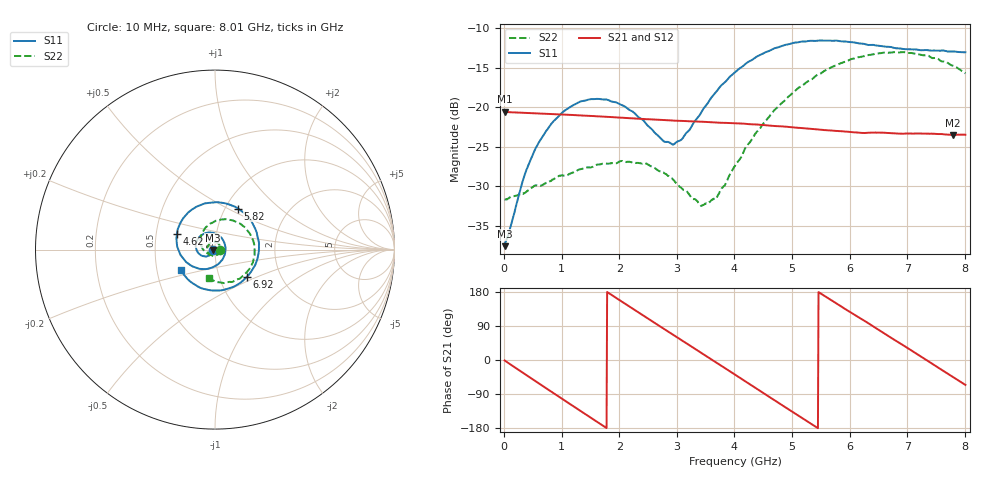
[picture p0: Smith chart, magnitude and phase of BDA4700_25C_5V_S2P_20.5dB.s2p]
!Agilent Technologies,E5071B,MY42404982,A.09.10
!Date: Mon Oct 20 13:36:39 2025
!Data & Calibration Information:
!Freq	S11:SOLT2(ON)	S21:SOLT2(ON)	S12:SOLT2(ON)	S22:SOLT2(ON)
# Hz S RI R 50
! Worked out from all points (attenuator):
!   801 points, 10 MHz to 8.01 GHz, reference 50 ohm
!   highest |S21| = -20.59 dB at 10 MHz (marker M1); lowest = -23.5 dB at 7.8 GHz (marker M2)
!   lowest |S11| = -37.6 dB at 10 MHz (marker M3), VSWR 1.03, Z = 48.7 - j0.149 ohm
!   |S11| at or under -10 dB: start of sweep to end of sweep
!   |S22| runs from -32.5 to -13.0 dB; largest |S21 - S12| = 0.00076
!   S11 on the Smith chart (normalised r, x): 10 MHz: 0.97, -0.00; 4.62 GHz: 0.64, +0.12; 5.82 GHz: 1.15, +0.56; 6.92 GHz: 1.36, -0.43; 8.01 GHz: 0.66, -0.16
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1e7  -0.0131 -0.00153  0.0935 -0.00199  0.0934 -0.00208  0.026 -0.000801
3.5e8  -0.0246 -0.0269  0.0745 -0.0541  0.0745 -0.0542  0.0222 -0.0178
5.7e8  -0.0427 -0.0376  0.0481 -0.0777  0.048 -0.0777  0.0143 -0.0286
8.8e8  -0.0763 -0.0328  0.000796 -0.0902  0.000764 -0.0904  -0.00699 -0.0347
1.35e9  -0.1077 0.0183  -0.0644 -0.0608  -0.0645 -0.0608  -0.0366 -0.0176
1.98e9  -0.052 0.0923  -0.0811 0.0287  -0.0811 0.0287  -0.0337 0.0294
2.46e9  0.0265 0.0746  -0.0331 0.0772  -0.0331 0.0772  -0.00135 0.0439
2.68e9  0.0511 0.0414  -0.00233 0.0832  -0.00236 0.0832  0.0141 0.0371
2.97e9  0.0567 -0.016  0.0369 0.0733  0.037 0.0732  0.0265 0.0206
3.44e9  -0.00467 -0.0948  0.0772 0.024  0.0773 0.024  0.0182 -0.0154
3.69e9  -0.064 -0.1081  0.0793 -0.01  0.0794 -0.0102  -0.000326 -0.0267
4.01e9  -0.1448 -0.0811  0.0618 -0.0494  0.0618 -0.0494  -0.0334 -0.0262
4.62e9  -0.2119 0.0852  -0.0117 -0.0755  -0.0117 -0.0755  -0.0797 0.0392
4.94e9  -0.1695 0.1844  -0.0483 -0.0573  -0.0483 -0.0575  -0.0712 0.0926
5.35e9  -0.0442 0.2591  -0.0718 -0.0124  -0.0718 -0.0126  -0.015 0.1498
5.82e9  0.1281 0.2285  -0.0575 0.0409  -0.0574 0.041  0.0908 0.1643
6.24e9  0.2301 0.1025  -0.0177 0.0664  -0.0171 0.0666  0.1802 0.1073
6.68e9  0.2305 -0.0698  0.0317 0.0609  0.0318 0.0609  0.2214 -0.00295
6.92e9  0.1792 -0.1499  0.0523 0.0435  0.0523 0.0432  0.2122 -0.0693
7.35e9  0.0285 -0.228  0.0679 -0.00202  0.068 -0.00217  0.1381 -0.1614
7.8e9  -0.139 -0.1772  0.047 -0.0473  0.0469 -0.0474  0.0171 -0.1818
8.01e9  -0.1902 -0.1157  0.0275 -0.061  0.0277 -0.0611  -0.033 -0.1601
